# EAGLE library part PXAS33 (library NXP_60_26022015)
XA 16-bit microcontroller 32 K/1 K OTP/ROM/ROMless, 8-channel 8-bit A/D, low voltage (2.7 V–5.5 V), I2C, 2 UARTs, 16 MB address range The XA-S3 device is a member of NXP Semiconductors’ XA (eXtended Architecture) family of high performance 16-bit single-chip microcontrollers. The XA-S3 device combines many powerful peripherals on one chip. With its high performance A/D converter, timers/counters, watchdog, Programmable Counter Array (PCA), I2C interface, dual UARTs, and multiple general purpose I/O ports, it is suited for general multipurpose high performance embedded control functions. AAL Eindhoven MK
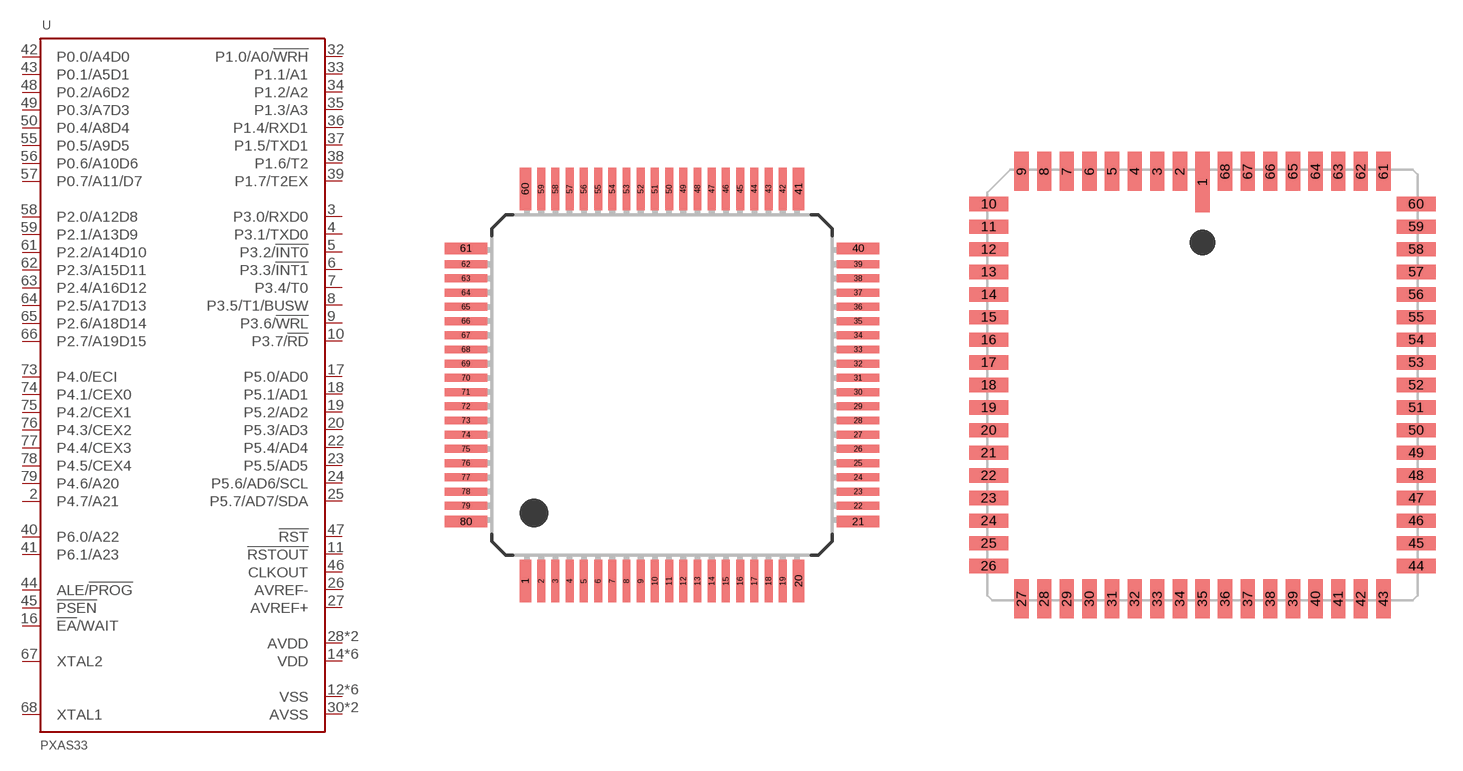
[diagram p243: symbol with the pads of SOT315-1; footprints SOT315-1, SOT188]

Designator prefix U

## PXAS33KBBE  [SOT315-1]
2  P4.7/A21
3  P3.0/RXD0
4  P3.1/TXD0
5  P3.2/!INT0!
6  P3.3/!INT1!
7  P3.4/T0
8  P3.5/T1/BUSW
9  P3.6/!WRL!
10  P3.7/!RD!
11  !RSTOUT!  out
12  VSS
13  VSS
14  VDD  pwr
15  VDD  pwr
16  !EA!/WAIT
17  P5.0/AD0
18  P5.1/AD1
19  P5.2/AD2
20  P5.3/AD3
22  P5.4/AD4
23  P5.5/AD5
24  P5.6/AD6/SCL
25  P5.7/AD7/SDA
26  AVREF-  pas
27  AVREF+  pas
28  AVDD  pwr
29  AVDD  pwr
30  AVSS  pwr
31  AVSS  pwr
32  P1.0/A0/!WRH!
33  P1.1/A1
34  P1.2/A2
35  P1.3/A3
36  P1.4/RXD1
37  P1.5/TXD1
38  P1.6/T2
39  P1.7/T2EX
40  P6.0/A22
41  P6.1/A23
42  P0.0/A4D0
43  P0.1/A5D1
44  ALE/!PROG!
45  !PSEN!  out
46  CLKOUT  out
47  !RST!  in
48  P0.2/A6D2
49  P0.3/A7D3
50  P0.4/A8D4
51  VDD  pwr
52  VDD  pwr
53  VSS
54  VSS
55  P0.5/A9D5
56  P0.6/A10D6
57  P0.7/A11/D7
58  P2.0/A12D8
59  P2.1/A13D9
61  P2.2/A14D10
62  P2.3/A15D11
63  P2.4/A16D12
64  P2.5/A17D13
65  P2.6/A18D14
66  P2.7/A19D15
67  XTAL2  out
68  XTAL1  in
69  VSS
70  VSS
71  VDD  pwr
72  VDD  pwr
73  P4.0/ECI
74  P4.1/CEX0
75  P4.2/CEX1
76  P4.3/CEX2
77  P4.4/CEX3
78  P4.5/CEX4
79  P4.6/A20

## PXAS33KBA  [SOT188]
1  VSS
2  VDD  pwr
3  P4.0/ECI
4  P4.1/CEX0
5  P4.2/CEX1
6  P4.3/CEX2
7  P4.4/CEX3
8  P4.5/CEX4
9  P4.6/A20
10  P4.7/A21
11  P3.0/RXD0
12  P3.1/TXD0
13  P3.2/!INT0!
14  P3.3/!INT1!
15  P3.4/T0
16  P3.5/T1/BUSW
17  P3.6/!WRL!
18  P3.7/!RD!
19  !RSTOUT!  out
20  VSS
21  VDD  pwr
22  !EA!/WAIT
23  P5.0/AD0
24  P5.1/AD1
25  P5.2/AD2
26  P5.3/AD3
27  P5.4/AD4
28  P5.5/AD5
29  P5.6/AD6/SCL
30  P5.7/AD7/SDA
31  AVREF-  pas
32  AVREF+  pas
33  AVDD  pwr
34  AVSS  pwr
35  P1.0/A0/!WRH!
36  P1.1/A1
37  P1.2/A2
38  P1.3/A3
39  P1.4/RXD1
40  P1.5/TXD1
41  P1.6/T2
42  P1.7/T2EX
43  P6.0/A22
44  P6.1/A23
45  P0.0/A4D0
46  P0.1/A5D1
47  ALE/!PROG!
48  !PSEN!  out
49  CLKOUT  out
50  !RST!  in
51  P0.2/A6D2
52  P0.3/A7D3
53  P0.4/A8D4
54  VDD  pwr
55  VSS
56  P0.5/A9D5
57  P0.6/A10D6
58  P0.7/A11/D7
59  P2.0/A12D8
60  P2.1/A13D9
61  P2.2/A14D10
62  P2.3/A15D11
63  P2.4/A16D12
64  P2.5/A17D13
65  P2.6/A18D14
66  P2.7/A19D15
67  XTAL2  out
68  XTAL1  in

## PXAS33KFA  [SOT188]
Pads as for SOT188

## PXAS33KFBE  [SOT315-1]
Pads as for SOT315-1

## Footprint SOT315-1 (pad centres in mm)
SOT315-1 LQFP80: plastic low profile quad flat package; 80 leads; body 12 x 12 x 1.4 mm JEDEC: MS-026 IEC: 136E15
smd 0.4 x 1.5: 1 -4.81,-6.9; 20 4.81,-6.9; 41 4.81,6.9; 60 -4.81,6.9
smd 0.28 x 1.5: 2 -4.25,-6.9; 3 -3.75,-6.9; 4 -3.25,-6.9; 5 -2.75,-6.9; 6 -2.25,-6.9; 7 -1.75,-6.9; 8 -1.25,-6.9; 9 -0.75,-6.9; 10 -0.25,-6.9; 11 0.25,-6.9; 12 0.75,-6.9; 13 1.25,-6.9; 14 1.75,-6.9; 15 2.25,-6.9; 16 2.75,-6.9; 17 3.25,-6.9; 18 3.75,-6.9; 19 4.25,-6.9; 42 4.25,6.9; 43 3.75,6.9; 44 3.25,6.9; 45 2.75,6.9; 46 2.25,6.9; 47 1.75,6.9; 48 1.25,6.9; 49 0.75,6.9; 50 0.25,6.9; 51 -0.25,6.9; 52 -0.75,6.9; 53 -1.25,6.9; 54 -1.75,6.9; 55 -2.25,6.9; 56 -2.75,6.9; 57 -3.25,6.9; 58 -3.75,6.9; 59 -4.25,6.9
smd 1.5 x 0.4: 21 6.9,-4.81; 40 6.9,4.81; 61 -6.9,4.81; 80 -6.9,-4.81
smd 1.5 x 0.28: 22 6.9,-4.25; 23 6.9,-3.75; 24 6.9,-3.25; 25 6.9,-2.75; 26 6.9,-2.25; 27 6.9,-1.75; 28 6.9,-1.25; 29 6.9,-0.75; 30 6.9,-0.25; 31 6.9,0.25; 32 6.9,0.75; 33 6.9,1.25; 34 6.9,1.75; 35 6.9,2.25; 36 6.9,2.75; 37 6.9,3.25; 38 6.9,3.75; 39 6.9,4.25; 62 -6.9,4.25; 63 -6.9,3.75; 64 -6.9,3.25; 65 -6.9,2.75; 66 -6.9,2.25; 67 -6.9,1.75; 68 -6.9,1.25; 69 -6.9,0.75; 70 -6.9,0.25; 71 -6.9,-0.25; 72 -6.9,-0.75; 73 -6.9,-1.25; 74 -6.9,-1.75; 75 -6.9,-2.25; 76 -6.9,-2.75; 77 -6.9,-3.25; 78 -6.9,-3.75; 79 -6.9,-4.25

## Footprint SOT188 (pad centres in mm)
SOT188 PLCC68: plastic leaded chip carrier; 68 leads JEDEC: MS-018 IEC: 112E10 JEITA: EDR-7319
smd 0.8 x 3.4: 1 0,11.4
smd 0.8 x 2.2: 2 -1.27,12; 3 -2.54,12; 4 -3.81,12; 5 -5.08,12; 6 -6.35,12; 7 -7.62,12; 8 -8.89,12; 9 -10.16,12; 27 -10.16,-12; 28 -8.89,-12; 29 -7.62,-12; 30 -6.35,-12; 31 -5.08,-12; 32 -3.81,-12; 33 -2.54,-12; 34 -1.27,-12; 35 0,-12; 36 1.27,-12; 37 2.54,-12; 38 3.81,-12; 39 5.08,-12; 40 6.35,-12; 41 7.62,-12; 42 8.89,-12; 43 10.16,-12; 61 10.16,12; 62 8.89,12; 63 7.62,12; 64 6.35,12; 65 5.08,12; 66 3.81,12; 67 2.54,12; 68 1.27,12
smd 2.2 x 0.8: 10 -12,10.16; 11 -12,8.89; 12 -12,7.62; 13 -12,6.35; 14 -12,5.08; 15 -12,3.81; 16 -12,2.54; 17 -12,1.27; 18 -12,0; 19 -12,-1.27; 20 -12,-2.54; 21 -12,-3.81; 22 -12,-5.08; 23 -12,-6.35; 24 -12,-7.62; 25 -12,-8.89; 26 -12,-10.16; 44 12,-10.16; 45 12,-8.89; 46 12,-7.62; 47 12,-6.35; 48 12,-5.08; 49 12,-3.81; 50 12,-2.54; 51 12,-1.27; 52 12,0; 53 12,1.27; 54 12,2.54; 55 12,3.81; 56 12,5.08; 57 12,6.35; 58 12,7.62; 59 12,8.89; 60 12,10.16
